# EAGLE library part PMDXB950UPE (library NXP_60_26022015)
20 V, dual P-channel Trench MOSFET Dual P-channel enhancement mode Field-Effect Transistor (FET) in a leadless ultra small DFN1010B-6 (SOT1216) Surface-Mounted Device (SMD) plastic package using Trench MOSFET technology. AAL Eindhoven MK
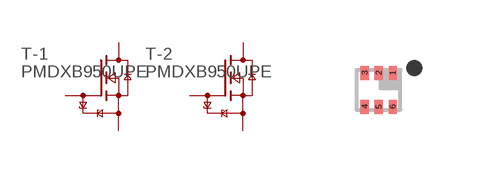
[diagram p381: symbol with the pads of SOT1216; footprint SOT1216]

Designator prefix T; gates -1=N-MOSFET-ESD -2=N-MOSFET-ESD

## PMDXB950UPE  [SOT1216]
1  -1:S  pas
2  -1:G  pas
3  -2:D  pas
4  -2:S  pas
5  -2:G  pas
6  -1:D  pas

## Footprint SOT1216 (pad centres in mm)
SOT1216 DFN1010B-6: plastic thermal enhanced ultra thin small outline package; no leads; 6 terminals; body: 1.1 x 1.0 x 0.37 mm JEDEC: -- IEC: -- JEITA: --date: 2013-11-06
smd 0.2 x 0.35: 1 0.35,0.425; 2 0,0.425; 3 -0.35,0.425; 4 -0.35,-0.425; 5 0,-0.425; 6 0.35,-0.425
